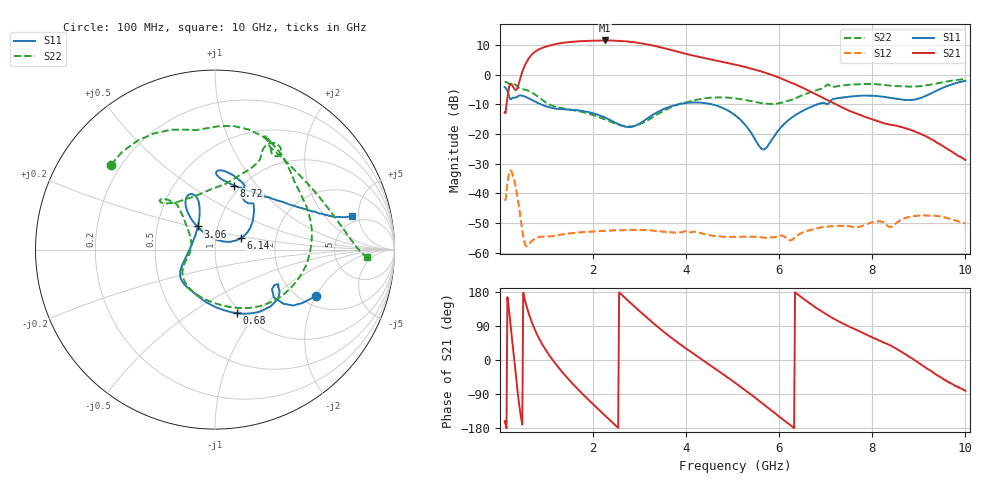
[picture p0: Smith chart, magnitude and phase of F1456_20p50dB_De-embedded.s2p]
! Integrated Device Technology
! Corporate Headquarters
! 6024 Silver Creek Valley Road
! San Jose, CA 95138  USA
! Phone:  1-408-284-8200
! Toll Free:  1-800-223-1366
! Webpage:  http://www.idt.com/
! Timing and RF Division
! 515 Groton Road, Suite 102
! Westford, MA 01886-6024
! Device:  F1456
! Description: 6-bit 0.5 dB Transmit Variable Gain Amplifier
! Frequency:  2100.0 -  2950.00 MHz
! Package:  6x6 mm Thin QFN Plastic Package: 28 pin
! State:  41
! Atten State:  20.5 dB
! Voltage:  +5.00 Volts
! Current:  216.962 mA
! Data:  The device was measured on a the F1455 evaluation board which has
!  individual transmission lines to the RF pins.  Data was collected
!  using a calibrated network analyzer.  The evaluation board was
!  de-embedded using a TRL calibration technique.
!  The reference plane is the edge of the package pin.
!  Pin  1 = CSb
!  Pin  2 = DATA
!  Pin  3 = CLK
!  Pin  4 = RSET
!  Pin  5 = GND
!  Pin  6 = RFIN  = Port 1
!  Pin  7 = GND
!  Pin  8 = NC
!  Pin  9 = NC
!  Pin 10 = NC
!  Pin 11 = NC
!  Pin 12 = NC
!  Pin 13 = NC
!  Pin 14 = /STBY
!  Pin 15 = GND
!  Pin 16 = RFOUT  = Port 2
!  Pin 17 = GND
!  Pin 18 = NC
!  Pin 19 = NC
!  Pin 20 = NC
!  Pin 21 = GND
!  Pin 22 = NC
!  Pin 23 = GND
!  Pin 24 = NC
!  Pin 25 = NC
!  Pin 26 = NC
!  Pin 27 = GND
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# GHz S dB R 50
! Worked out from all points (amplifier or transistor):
!   496 points, 100 MHz to 10 GHz, reference 50 ohm
!   highest |S21| = 11.5 dB at 2.26 GHz (marker M1)
!   |S21| within 3 dB of that: 834.6 MHz to 3.627 GHz (2.793 GHz wide, 125 % of centre)
!   unconditionally stable (mu >= 1): start of sweep to end of sweep
!   at 1.74 GHz: K = 55.15, MAG = 11.8 dB, |S12| = -53.1 dB
!   at 5.06 GHz: K = 148.77, MAG = 4.3 dB, |S12| = -54.7 dB
!   at 10 GHz: K = 479.73, MAG = -19.1 dB, |S12| = -50.1 dB
!   S11 on the Smith chart (normalised r, x): 100 MHz: 2.37, -2.00; 680 MHz: 0.96, -0.79; 3.06 GHz: 0.80, +0.21; 6.14 GHz: 1.32, +0.17; 8.72 GHz: 0.93, +0.77; 10 GHz: 4.20, +4.08
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0.1  -4.16 -25.0  -12.74 -161.2  -42.29 49.2  -2.53 140.8
0.22  -8.25 -34.8  -3.17 101.6  -32.30 -51.0  -3.43 99.1
0.3  -7.77 -30.6  -4.58 10.1  -35.19 -135.1  -3.16 74.7
0.42  -7.06 -37.4  -2.20 -124.6  -45.71 141.8  -4.66 41.2
0.54  -7.39 -54.0  3.27 156.4  -57.21 139.7  -5.11 16.5
0.68  -8.50 -70.8  6.66 101.3  -56.12 145.9  -5.98 -15.1
0.86  -9.88 -89.4  8.67 52.1  -54.62 112.6  -7.94 -52.0
1.16  -11.37 -114.4  10.13 -4.4  -54.35 75.9  -10.68 -94.1
1.48  -11.78 -131.9  10.93 -51.8  -53.49 51.8  -11.76 -123.2
1.76  -12.22 -142.3  11.25 -87.9  -53.07 35.1  -12.58 -139.5
2.26  -14.49 -158.5  11.48 -147.0  -52.59 11.5  -15.14 -158.8
2.64  -17.32 173.5  11.28 169.4  -52.38 -6.1  -17.25 -177.0
3.06  -15.90 126.3  10.45 122.3  -52.26 -26.1  -16.37 154.1
3.4  -12.51 111.2  9.37 86.4  -52.64 -41.5  -13.28 138.4
4.1  -9.42 113.4  6.57 21.7  -53.07 -72.6  -8.95 131.6
5.06  -13.77 128.1  3.32 -60.7  -54.65 -119.8  -8.02 138.7
5.66  -25.16 72.1  0.83 -116.5  -54.86 -157.7  -9.71 122.0
6.14  -16.14 23.8  -1.99 -162.8  -54.91 167.8  -9.09 87.2
6.7  -10.77 41.9  -5.96 145.6  -52.22 146.7  -5.79 65.1
8.36  -7.74 87.9  -16.77 40.1  -51.29 71.7  -3.71 62.4
8.72  -8.58 73.3  -18.14 14.8  -48.28 69.7  -4.01 50.2
10  -2.11 13.8  -28.73 -81.6  -50.10 -22.0  -1.46 -2.6
